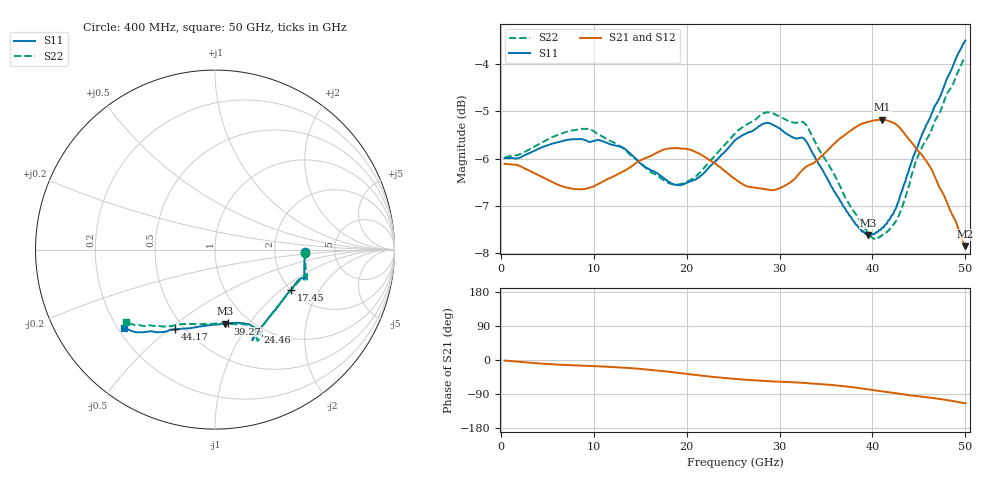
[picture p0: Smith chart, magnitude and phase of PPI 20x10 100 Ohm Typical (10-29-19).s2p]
!Keysight Technologies,N5227A,US56070614,A.10.47.06
!Date:	11/6/2019
!Correction
!S11(Full 2 Port(1,2))
!S21(Full 2 Port(1,2))
!S12(Full 2 Port(1,2))
!S22(Full 2 Port(1,2))
!S2P File: Measurements: S11, S21, S12, S22
# GHz S  dB  R 50
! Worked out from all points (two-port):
!   801 points, 400 MHz to 50 GHz, reference 50 ohm
!   highest |S21| = -5.17 dB at 41.07 GHz (marker M1); lowest = -7.9 dB at 50 GHz (marker M2)
!   |S21| within 3 dB of the highest: start of sweep to end of sweep
!   lowest |S11| = -7.6 dB at 39.52 GHz (marker M3), VSWR 2.42, Z = 39.1 - j39 ohm
!   |S11| at or under -10 dB: nowhere
!   |S22| runs from -7.7 to -3.8 dB; largest |S21 - S12| = 0.0022
!   S11 on the Smith chart (normalised r, x): 400 MHz: 3.01, -0.13; 17.45 GHz: 2.02, -1.17; 24.46 GHz: 0.93, -1.16; 39.27 GHz: 0.80, -0.80; 44.17 GHz: 0.45, -0.53; 50 GHz: 0.22, -0.36
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0.4  -5.99 -1.8  -6.11 -1.5  -6.11 -1.5  -5.98 -1.9
4.55  -5.75 -15.3  -6.40 -9.7  -6.40 -9.8  -5.64 -13.8
6.6  -5.63 -17.5  -6.59 -12.6  -6.59 -12.7  -5.46 -16.4
8.71  -5.59 -16.9  -6.65 -14.9  -6.66 -14.9  -5.37 -17.5
12.06  -5.71 -17.8  -6.38 -18.6  -6.39 -18.6  -5.65 -16.1
14.66  -6.03 -19.4  -6.08 -22.7  -6.08 -22.8  -6.03 -20.4
16.95  -6.33 -25.7  -5.86 -27.8  -5.86 -27.9  -6.38 -28.7
17.45  -6.40 -27.8  -5.81 -29.2  -5.82 -29.3  -6.45 -31.0
21.29  -6.40 -48.8  -5.89 -40.4  -5.90 -40.5  -6.32 -51.6
24.46  -5.78 -62.4  -6.32 -48.5  -6.33 -48.6  -5.63 -62.9
25.2  -5.61 -64.4  -6.43 -50.1  -6.44 -50.2  -5.47 -64.1
28.86  -5.25 -67.6  -6.66 -56.0  -6.67 -56.1  -5.02 -64.8
32.21  -5.56 -63.9  -6.29 -59.7  -6.30 -59.8  -5.22 -61.1
33.51  -5.87 -63.8  -6.11 -62.4  -6.12 -62.5  -5.52 -61.7
36.24  -6.80 -65.7  -5.62 -67.5  -5.63 -67.5  -6.47 -64.1
39.27  -7.59 -79.9  -5.23 -76.6  -5.24 -76.7  -7.50 -79.1
39.52  -7.62 -82.0  -5.22 -77.5  -5.23 -77.6  -7.58 -81.2
41.07  -7.46 -94.7  -5.17 -82.8  -5.18 -83.0  -7.62 -94.7
41.75  -7.31 -98.8  -5.20 -84.9  -5.21 -85.1  -7.52 -99.7
44.17  -6.10 -116.4  -5.65 -93.6  -5.66 -93.8  -6.38 -118.3
48.64  -4.05 -132.8  -7.21 -108.2  -7.22 -108.4  -4.43 -135.6
50  -3.50 -139.2  -7.86 -114.2  -7.86 -114.5  -3.84 -140.8
